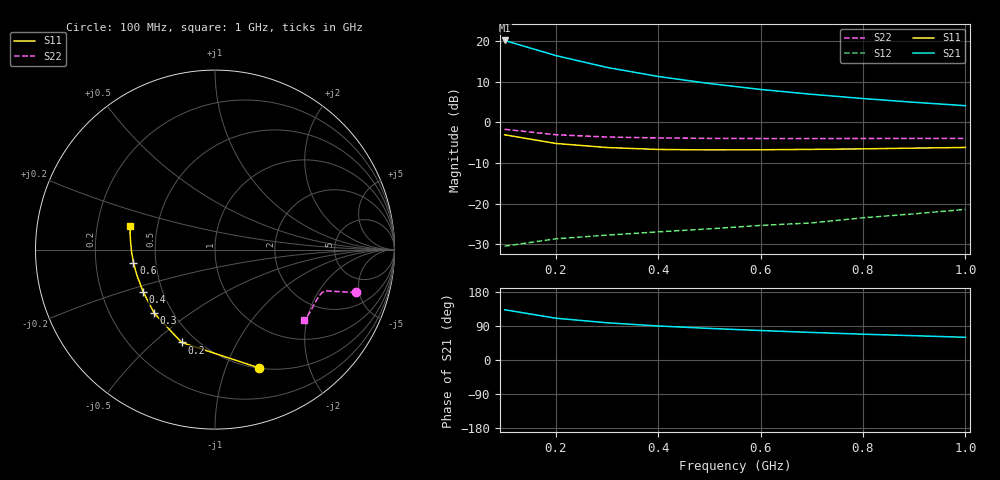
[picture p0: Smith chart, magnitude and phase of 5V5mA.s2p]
#  HZ  S  MA  R  50.0000
! Device:15GN03CA
! "! Bias:VCE=5V, IC=5mA  "
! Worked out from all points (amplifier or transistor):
!   10 points, 100 MHz to 1 GHz, reference 50 ohm
!   highest |S21| = 20.1 dB at 100 MHz (marker M1)
!   |S21| within 3 dB of that: start of sweep to 180.7 MHz
!   unconditionally stable (mu >= 1): 285 MHz to end of sweep
!   at 200 MHz: K = 0.76, MSG = 22.5 dB, |S12| = -28.6 dB
!   at 600 MHz: K = 1.53, MAG = 12.4 dB, |S12| = -25.4 dB
!   at 1 GHz: K = 1.43, MAG = 8.9 dB, |S12| = -21.4 dB
!   S11 on the Smith chart (normalised r, x): 100 MHz: 0.50, -1.31; 200 MHz: 0.42, -0.62; 300 MHz: 0.40, -0.37; 400 MHz: 0.39, -0.23; 600 MHz: 0.37, -0.07; 1 GHz: 0.35, +0.12
1e8  0.703 -69.6  10.16 132.6  0.03 54.5  0.821 -16.9
2e8  0.55 -109.8  6.625 110.3  0.037 43.2  0.704 -19.3
3e8  0.49 -133.8  4.733 98.2  0.041 44.9  0.66 -20.4
4e8  0.464 -149.7  3.666 89.8  0.045 49.1  0.643 -21.8
5e8  0.458 -161.7  3.003 83.3  0.049 56.1  0.635 -24.0
6e8  0.46 -171.0  2.537 77.8  0.054 60.2  0.632 -26.5
7e8  0.465 -178.5  2.212 72.7  0.058 65.9  0.631 -29.1
8e8  0.472 174.9  1.962 68.1  0.067 71.0  0.633 -32.1
9e8  0.482 169.1  1.764 64.1  0.075 76.6  0.634 -35.3
1e9  0.491 164.2  1.602 59.9  0.085 79.0  0.635 -38.3
